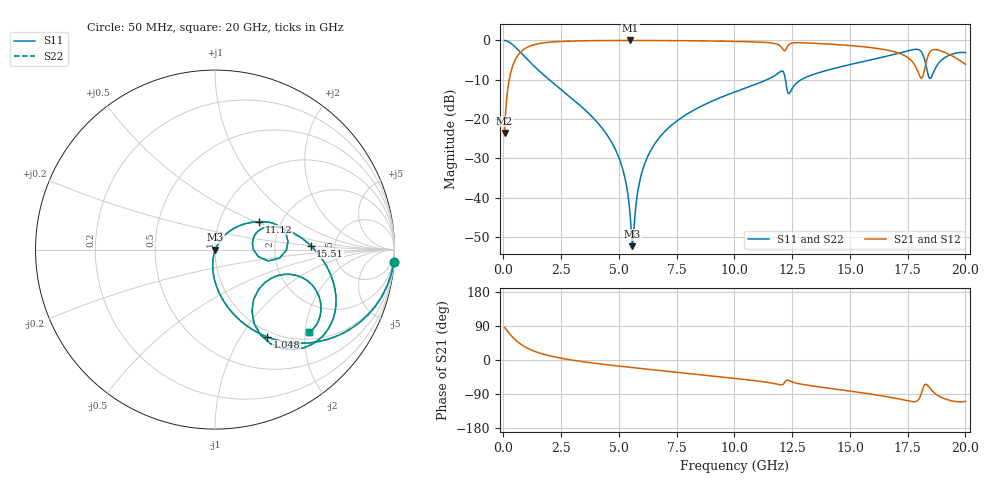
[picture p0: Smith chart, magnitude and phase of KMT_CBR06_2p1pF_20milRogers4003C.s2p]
! Data measured by Modelithics Inc. support@modelithics.com 813-866-6335
! KEMET CBR0603 2.1pF, Pad Width= 0.851mm, Pad Length= 0.64mm, Pad Gap= 0.62mm, 20mil Rogers 4003C substrate Data, January 2022
# hz S ma R 50
! 2 Port Network Data from SP1.SP block
! freq  magS11  angS11  magS21  angS21  magS12  angS12  magS22  angS22
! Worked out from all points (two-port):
!   401 points, 50 MHz to 20 GHz, reference 50 ohm
!   highest |S21| = -0.02 dB at 5.486 GHz (marker M1); lowest = -23.5 dB at 50 MHz (marker M2)
!   |S21| within 3 dB of the highest: 736.4 MHz to 17 GHz (16.27 GHz wide, 183 % of centre); 18.46 GHz to 19.09 GHz (634 MHz wide, 3.38 % of centre)
!   lowest |S11| = -52.3 dB at 5.586 GHz (marker M3), VSWR 1.00, Z = 50.2 - j0.103 ohm
!   |S11| at or under -10 dB: 1.983 GHz to 11.41 GHz (9.423 GHz wide, 141 % of centre); 12.21 GHz to 12.89 GHz (679.7 MHz wide, 5.42 % of centre)
!   |S22| runs from -52.3 to 0.0 dB; largest |S21 - S12| = 0
!   S11 on the Smith chart (normalised r, x): 50 MHz: 1, -29; 1.048 GHz: 0.92, -1.32; 11.12 GHz: 1.55, +0.53; 15.51 GHz: 3.27, +0.21; 20 GHz: 1.17, -2.11
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5e7  0.9978 -4.0  0.06668 86.0  0.06668 86.0  0.9978 -4.0
3.99125e8  0.881 -29.6  0.4721 60.3  0.4721 60.3  0.881 -29.6
1.0475e9  0.5682 -59.0  0.8215 30.8  0.8215 30.8  0.5682 -59.0
3.391625e9  0.1427 -93.2  0.9876 -4.0  0.9876 -4.0  0.1427 -93.2
4.887875e9  0.03876 -102.0  0.9968 -15.4  0.9968 -15.4  0.03876 -102.0
5.286875e9  0.01641 -99.8  0.9973 -18.1  0.9973 -18.1  0.01641 -99.8
5.486375e9  0.005991 -85.8  0.9974 -19.4  0.9974 -19.4  0.005991 -85.8
5.586125e9  0.002431 -25.0  0.9974 -20.1  0.9974 -20.1  0.002431 -25.0
6.035e9  0.02303 60.7  0.997 -23.0  0.997 -23.0  0.02303 60.7
6.73325e9  0.05742 59.9  0.9955 -27.4  0.9955 -27.4  0.05742 59.9
1.0025e10  0.2218 40.5  0.9707 -48.4  0.9707 -48.4  0.2218 40.5
1.112225e10  0.2919 32.3  0.9493 -56.4  0.9493 -56.4  0.2919 32.3
1.22195e10  0.3029 -12.0  0.7567 -55.1  0.7567 -55.1  0.3029 -12.0
1.2419e10  0.2215 16.1  0.9091 -56.0  0.9091 -56.0  0.2215 16.1
1.336662e10  0.3651 20.1  0.921 -68.4  0.921 -68.4  0.3651 20.1
1.551125e10  0.5333 2.4  0.834 -86.4  0.834 -86.4  0.5333 2.4
1.670825e10  0.6416 -10.1  0.7426 -97.9  0.7426 -97.9  0.6416 -10.1
1.775562e10  0.765 -31.3  0.5111 -110.1  0.5111 -110.1  0.765 -31.3
1.810475e10  0.7073 -52.0  0.3307 -85.7  0.3307 -85.7  0.7073 -52.0
1.835412e10  0.3989 -59.0  0.6024 -66.3  0.6024 -66.3  0.3989 -59.0
1.875312e10  0.4706 -17.6  0.7608 -91.5  0.7608 -91.5  0.4706 -17.6
2e10  0.699 -41.2  0.4974 -109.0  0.4974 -109.0  0.699 -41.2
